// TwinCAT 3 PLC project CPUTemperture
// ProgramVersion: 3.1.4022.0
// libraries:
//   Tc2_MDP, * (Beckhoff Automation GmbH)
//   Tc2_Standard, * (Beckhoff Automation GmbH)
//   Tc2_System, * (Beckhoff Automation GmbH)
//   Tc3_Module, * (Beckhoff Automation GmbH)
// project tree:
//   DUTs/ E_State.TcDUT
//   / PlcTask.TcTTO
//   POUs/ MAIN.TcPOU

CONFIGURATION CPUTemperture
    RESOURCE PLC ON TwinCAT3
        TASK PlcTask(INTERVAL := T#10ms, PRIORITY := 20);
        PROGRAM MAIN WITH PlcTask : MAIN;
    END_RESOURCE
END_CONFIGURATION

// ---- DUTs/E_State.TcDUT

TYPE E_State :
(
    eState_InitiateStateMachine    :=0, 
	eState_ReadCPUTempertureInit   :=20, 
    eState_ReadCPUTemperture       :=21,    
    eState_IdleState               :=100   
);
END_TYPE

// ---- POUs/MAIN.TcPOU
PROGRAM MAIN
VAR
	//内部使用
    sAmsNetId           : STRING := '';        //控制器的NETID, 本地的NETID可以为空       
    eState              : E_State;          
    bRestart            : BOOL;                //重启触发位       
    uData               : UINT;                  
    stMDP_Addr          : ST_MDP_Addr;        //包括MDP的所有地址参数      
    fbReadMDPElement    : FB_MDP_ReadElement; //读取MDP参数的功能块
//输出变量
    bError              : BOOL;              
    nErrID              : UDINT;                           
	iCpuTemperture      : UINT;              //CPU温度
END_VAR

//该程序实可以读取CPU的实时温度

//初始化PLC参数,把FB_MDP_ReadElement功能的执行标志位复位，让输出变量bError,nErrID复位;
CASE eState OF
    eState_InitiateStateMachine:             
    fbReadMDPElement(bExecute := FALSE); 
    bError:=FALSE;
    nErrID:=0;  
    eState := eState_ReadCPUTempertureInit;  //通过CASE语句，跳转到eState_ReadCPUTempertureInit步  


//设置指要读取的地址
//CPU的温度这个参数在MDP列表具体位置
//地区：eMDP_Area_ConfigArea
//table ID为1
//subIndex为3
    eState_ReadCPUTempertureInit:    
        stMDP_Addr.nArea    := INT_TO_BYTE(eMDP_Area_ConfigArea); 
        stMDP_Addr.nTableId := 1;              
        stMDP_Addr.nSubIdx  := 03;                                 
//执行fbReadMDPElement读取CPU温度      
        fbReadMDPElement(
            bExecute    := TRUE,             
            eModuleType := eMDP_ModT_CPU,   //模块类型为CPU           
            stMDP_Addr  := stMDP_Addr,          
            iModIdx     := 0,              //默认为0   
            pDstBuf     := ADR(uData),    //CPU温度参数保存在uData变量中     
            cbDstBufLen := SIZEOF(uData),      
            sAmsNetId   := sAmsNetId,          
            );                                

       eState := eState_ReadCPUTemperture;  //通过Case语句，跳转到eState_ReadCPUTemperture步

//该步实现把读到的CPU温度传送给iCpuTemperture
//并且通过fbReadMDPElement.bError判断执行哪步            
    eState_ReadCPUTemperture:              //把FB_MDP_ReadElement功能的执行标志位复位
        fbReadMDPElement(bExecute := FALSE);                                               
//通过fbReadMDPElement.bError判断，是否功能块执行报错
//如果报错，跳转到eState_IdleState
//如果没有报错，则会跳到eState_ReadCPUTempertureInit,重新循环读取CPU的温度
        IF NOT fbReadMDPElement.bBusy THEN     
            IF fbReadMDPElement.bError THEN   
                bError    := TRUE;            
                nErrID    := fbReadMDPElement.nErrID;                                  
                eState    := eState_IdleState; 
            ELSE                               
                bError    := FALSE;           
                iCpuTemperture := uData;           
                eState    := eState_ReadCPUTempertureInit; 
            END_IF
        END_IF

 //当fbReadMDPElement报错的时候，通过触发 bRestart来实现复位 
     eState_IdleState:                        
         IF bRestart THEN                      
            eState := eState_InitiateStateMachine;
    END_IF    
ELSE
    eState := eState_IdleState;                 
END_CASE

END_PROGRAM
